FUNCTION "Schrittkette16" : VOID
TITLE =Schrittkette
//KNOW_HOW_PROTECT
//
//Stand: Dezember 2006 /
//by R.Kleißler /
// Achtung in der Schrittkette ist das Schieberegister FC121 integriert,
// FC121 mit in die CPU kopieren.
AUTHOR : 'Kleißler'
VERSION : 0.1


VAR_INPUT
  Takt : BOOL ;
  IN0 : BOOL ;
  IN1 : BOOL ;
  IN2 : BOOL ;
  IN3 : BOOL ;
  IN4 : BOOL ;
  IN5 : BOOL ;
  IN6 : BOOL ;
  IN7 : BOOL ;
  IN8 : BOOL ;
  IN9 : BOOL ;
  IN10 : BOOL ;
  IN11 : BOOL ;
  IN12 : BOOL ;
  IN13 : BOOL ;
  IN14 : BOOL ;
  IN15 : BOOL ;
  Reset : BOOL ;
END_VAR
VAR_OUTPUT
  OUT0 : BOOL ;
  OUT1 : BOOL ;
  OUT2 : BOOL ;
  OUT3 : BOOL ;
  OUT4 : BOOL ;
  OUT5 : BOOL ;
  OUT6 : BOOL ;
  OUT7 : BOOL ;
  OUT8 : BOOL ;
  OUT9 : BOOL ;
  OUT10 : BOOL ;
  OUT11 : BOOL ;
  OUT12 : BOOL ;
  OUT13 : BOOL ;
  OUT14 : BOOL ;
  OUT15 : BOOL ;
END_VAR
VAR_IN_OUT
  HMWord : WORD ;
END_VAR
VAR_TEMP
  HMBit : BOOL ;
  HMBit_1 : BOOL ;
END_VAR
BEGIN
NETWORK
TITLE =Schieberegister
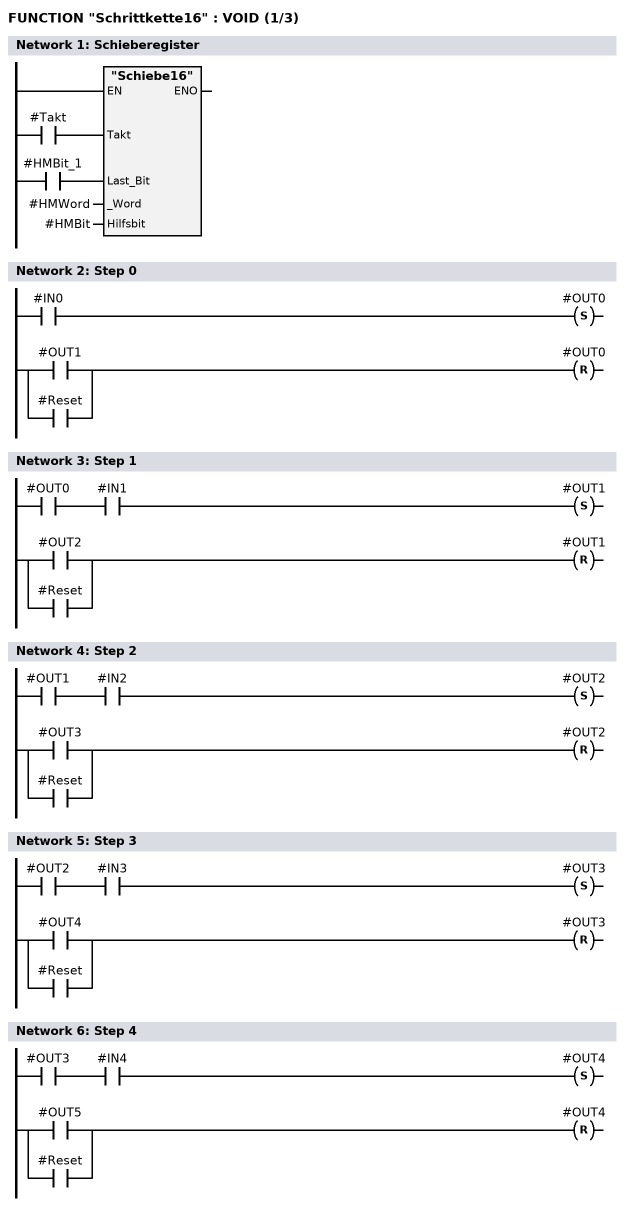
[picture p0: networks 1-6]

      U     #Takt;
      =     L      1.0;
      BLD   103;
      U     #HMBit_1;
      =     L      1.1;
      BLD   103;
      CALL "Schiebe16" (
           Takt                     := L      1.0,
           Last_Bit                 := L      1.1,
           _Word                    := #HMWord,
           Hilfsbit                 := #HMBit);
      NOP   0;
NETWORK
TITLE =Step 0

      U     #IN0;
      S     #OUT0;
      U(    ;
      O     #OUT1;
      O     #Reset;
      )     ;
      R     #OUT0;
      NOP   0;
NETWORK
TITLE =Step 1

      U     #OUT0;
      U     #IN1;
      S     #OUT1;
      U(    ;
      O     #OUT2;
      O     #Reset;
      )     ;
      R     #OUT1;
      NOP   0;
NETWORK
TITLE =Step 2

      U     #OUT1;
      U     #IN2;
      S     #OUT2;
      U(    ;
      O     #OUT3;
      O     #Reset;
      )     ;
      R     #OUT2;
      NOP   0;
NETWORK
TITLE =Step 3

      U     #OUT2;
      U     #IN3;
      S     #OUT3;
      U(    ;
      O     #OUT4;
      O     #Reset;
      )     ;
      R     #OUT3;
      NOP   0;
NETWORK
TITLE =Step 4

      U     #OUT3;
      U     #IN4;
      S     #OUT4;
      U(    ;
      O     #OUT5;
      O     #Reset;
      )     ;
      R     #OUT4;
      NOP   0;
NETWORK
TITLE =Step 5
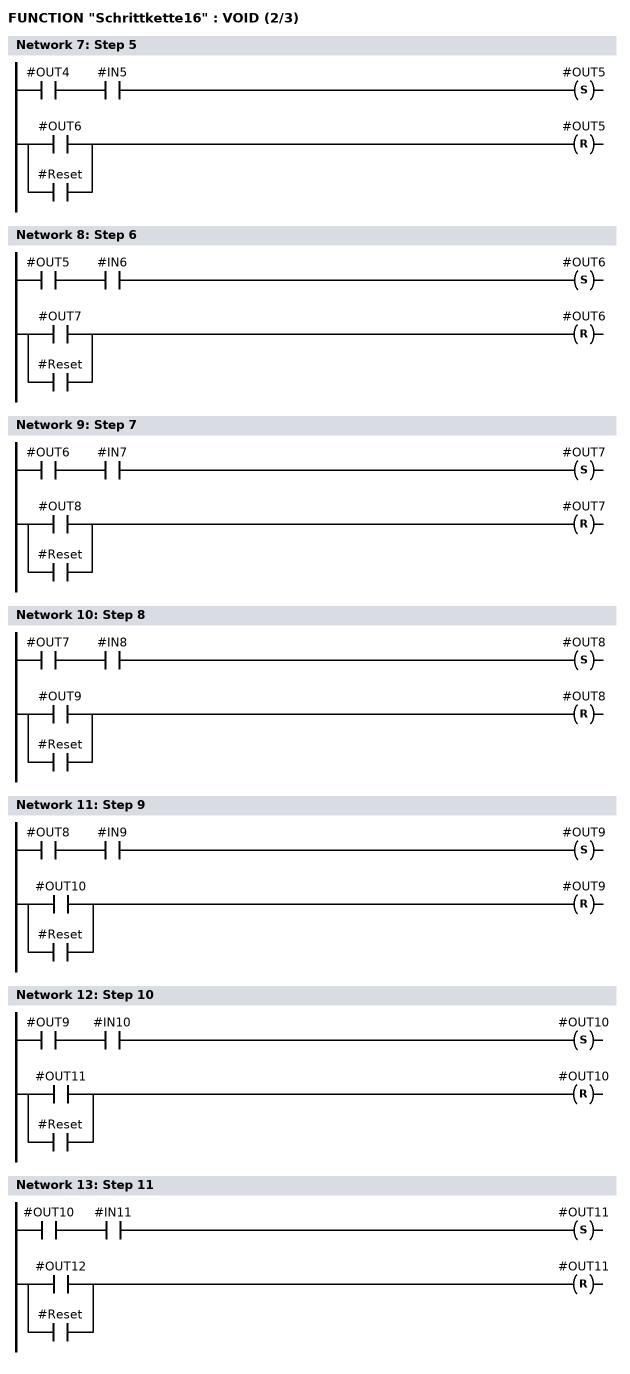
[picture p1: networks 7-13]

      U     #OUT4;
      U     #IN5;
      S     #OUT5;
      U(    ;
      O     #OUT6;
      O     #Reset;
      )     ;
      R     #OUT5;
      NOP   0;
NETWORK
TITLE =Step 6

      U     #OUT5;
      U     #IN6;
      S     #OUT6;
      U(    ;
      O     #OUT7;
      O     #Reset;
      )     ;
      R     #OUT6;
      NOP   0;
NETWORK
TITLE =Step 7

      U     #OUT6;
      U     #IN7;
      S     #OUT7;
      U(    ;
      O     #OUT8;
      O     #Reset;
      )     ;
      R     #OUT7;
      NOP   0;
NETWORK
TITLE =Step 8

      U     #OUT7;
      U     #IN8;
      S     #OUT8;
      U(    ;
      O     #OUT9;
      O     #Reset;
      )     ;
      R     #OUT8;
      NOP   0;
NETWORK
TITLE =Step 9

      U     #OUT8;
      U     #IN9;
      S     #OUT9;
      U(    ;
      O     #OUT10;
      O     #Reset;
      )     ;
      R     #OUT9;
      NOP   0;
NETWORK
TITLE =Step 10

      U     #OUT9;
      U     #IN10;
      S     #OUT10;
      U(    ;
      O     #OUT11;
      O     #Reset;
      )     ;
      R     #OUT10;
      NOP   0;
NETWORK
TITLE =Step 11

      U     #OUT10;
      U     #IN11;
      S     #OUT11;
      U(    ;
      O     #OUT12;
      O     #Reset;
      )     ;
      R     #OUT11;
      NOP   0;
NETWORK
TITLE =Step 12
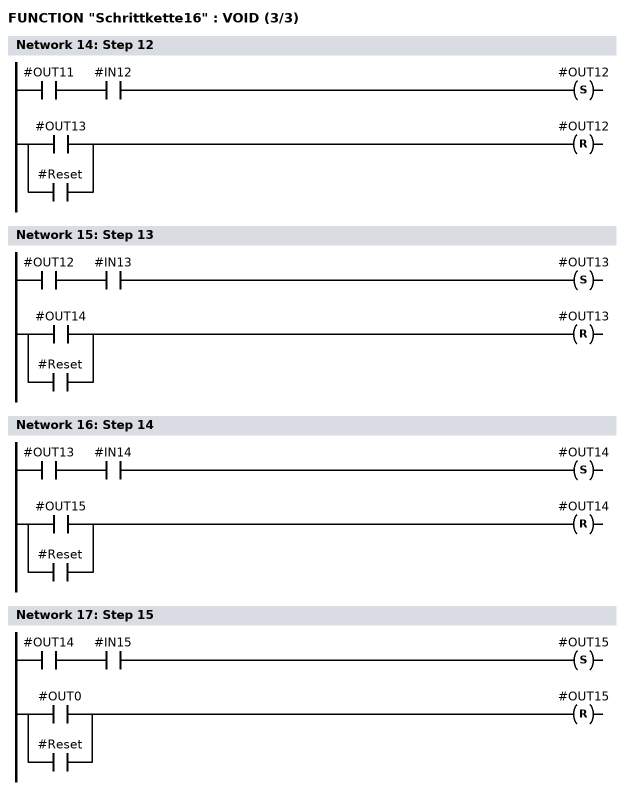
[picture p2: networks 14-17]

      U     #OUT11;
      U     #IN12;
      S     #OUT12;
      U(    ;
      O     #OUT13;
      O     #Reset;
      )     ;
      R     #OUT12;
      NOP   0;
NETWORK
TITLE =Step 13
//
//
      U     #OUT12;
      U     #IN13;
      S     #OUT13;
      U(    ;
      O     #OUT14;
      O     #Reset;
      )     ;
      R     #OUT13;
      NOP   0;
NETWORK
TITLE =Step 14
//
//
      U     #OUT13;
      U     #IN14;
      S     #OUT14;
      U(    ;
      O     #OUT15;
      O     #Reset;
      )     ;
      R     #OUT14;
      NOP   0;
NETWORK
TITLE =Step 15
//
//
//
      U     #OUT14;
      U     #IN15;
      S     #OUT15;
      U(    ;
      O     #OUT0;
      O     #Reset;
      )     ;
      R     #OUT15;
      NOP   0;
END_FUNCTION

